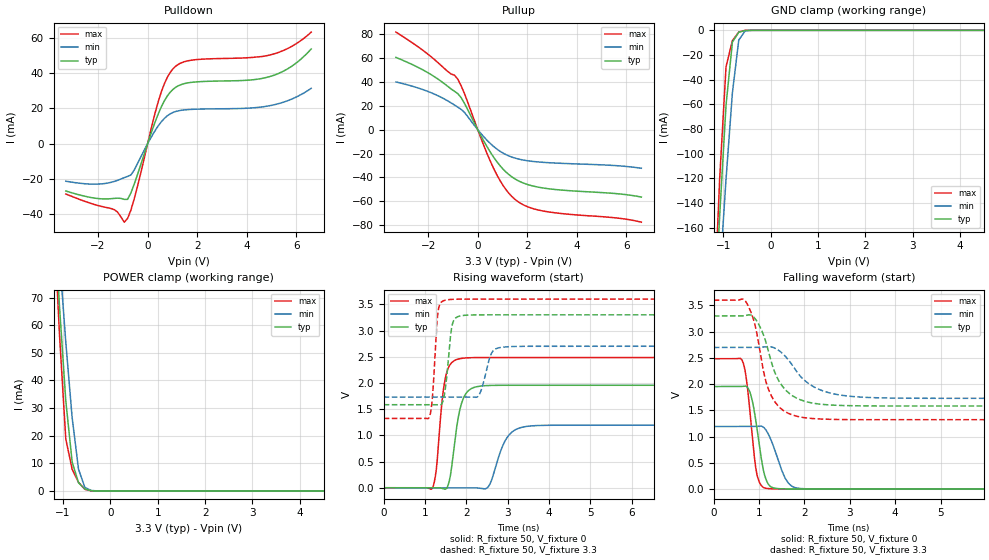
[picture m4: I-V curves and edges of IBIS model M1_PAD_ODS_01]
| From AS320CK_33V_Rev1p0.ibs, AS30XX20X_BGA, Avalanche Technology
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[Model] M1_PAD_ODS_01
Model_type I/O
Enable   Active-High
Vinl  =  0.8
Vinh  =  2.2
Vmeas =  1.65
Cref  =  30e-12
| Capacitance  typ   min   max
C_comp   1.518728e-12   1.426995e-12   1.652439e-12
| Variables   typ   min   max
[GND Clamp Reference]   0   0   0
[POWER Clamp Reference]   3.3   2.7   3.6
[Pulldown Reference]   0   0   0
[Pullup Reference]   3.3   2.7   3.6
[Temperature Range]   25   125   -40
[Voltage Range]   3.3   2.7   3.6
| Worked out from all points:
|   slope of the pulldown table from 0 to 0.495 V, typ, clamps not added: 26.1 ohm
|   slope of the pullup table from 0 to 0.495 V, typ, clamps not added: 27 ohm
|   GND clamp passes 1 mA (typ) near -0.62 V on its own axis
|   POWER clamp passes 1 mA (typ) near -0.56 V on its own axis
|   falling waveform, R_fixture 50, V_fixture 0: 20-80 % time 210ps typ, 304ps min, 176ps max; typ from 1.96 V to 0 V
|   falling waveform, R_fixture 50, V_fixture 3.3: 20-80 % time 456ps typ, 660ps min, 366ps max; typ from 3.3 V to 1.58 V
|   rising waveform, R_fixture 50, V_fixture 0: 20-80 % time 224ps typ, 335ps min, 176ps max; typ from 0 V to 1.96 V
|   rising waveform, R_fixture 50, V_fixture 3.3: 20-80 % time 128ps typ, 193ps min, 104ps max; typ from 1.58 V to 3.3 V
[GND Clamp]
| Voltage   I(typ)   I(min)   I(max)
-3.3V     -1.961A    -1.697A    -2.357A
-1.21V    -250.6mA   -283.7mA   -242.3mA
-1.076V   -150.5mA   -200.1mA   -120.5mA
-941.4mV  -60.74mA   -120.8mA   -29.57mA
-806.9mV  -9.575mA   -50.7mA    -8.297mA
-672.4mV  -1.554mA   -7.862mA   -1.403mA
-537.9mV  -68.54uA   -503.1uA   -16.86uA
-403.4mV  -562.8nA   -18.5uA    -33.35nA
6.6V      0A         0A         0A
[POWER Clamp]
| Voltage   I(typ)   I(min)   I(max)
-3.3V     772.3mA    673.3mA    930.5mA
-1.21V    105.9mA    117.6mA    104.6mA
-1.076V   67.34mA    85.06mA    57.16mA
-941.4mV  32.71mA    53.93mA    18.82mA
-806.9mV  10.48mA    26.53mA    7.848mA
-672.4mV  2.975mA    7.856mA    3.108mA
-537.9mV  710.9uA    1.248mA    573.1uA
-403.4mV  60.69uA    160.8uA    9.187uA
-269mV    142.4nA    6.118uA    23.26nA
6.6V      0A         0A         0A
[Pulldown]
| Voltage   I(typ)   I(min)   I(max)
-3.3V     -26.75mA   -21.23mA   -28.47mA
-1.345V   -30.95mA   -21.36mA   -37.3mA
-941.4mV  -31.51mA   -19.19mA   -44.41mA
-806.9mV  -31.48mA   -18.5mA    -42.27mA
-537.9mV  -22.81mA   -14.83mA   -31.1mA
455.2mV   17.74mA    10.61mA    25.04mA
682.8mV   24.44mA    14.41mA    34.16mA
1.024V    30.75mA    17.67mA    42.38mA
1.821V    34.78mA    19.45mA    47.35mA
4.914V    37.93mA    21.47mA    50.14mA
5.783V    43.54mA    25.06mA    54.82mA
6.6V      53.61mA    31.34mA    63.15mA
[Pullup]
| Voltage   I(typ)   I(min)   I(max)
-3.3V     60.72mA    40.13mA    81.98mA
-1.883V   46.28mA    31.07mA    61.29mA
-806.9mV  30.37mA    18.97mA    42.5mA
-537.9mV  22.23mA    14.55mA    30.47mA
227.6mV   -8.879mA   -5.576mA   -12.4mA
682.8mV   -24.3mA    -14.8mA    -34.27mA
1.138V    -35.52mA   -20.92mA   -50.3mA
1.593V    -42.39mA   -24.36mA   -59.94mA
2.048V    -46.27mA   -26.18mA   -65mA
2.731V    -49.23mA   -27.53mA   -68.61mA
5.659V    -53.82mA   -30.29mA   -74.27mA
6.6V      -56.57mA   -32.36mA   -77.67mA
[Ramp]
dV/dt_r   1.17342/0.223753n  0.716081/0.335063n  1.491/0.176015n
dV/dt_f   1.02933/0.456193n  0.581576/0.660479n  1.3662/0.365831n
R_load = 50
[Falling Waveform]
R_fixture = 50
V_fixture = 0
V_fixture_min = 0
V_fixture_max = 0
| Time   V(typ)   V(min)   V(max)
0s        1.956V     1.193V     2.485V
633.4ps   1.958V     1.194V     2.44V
712ps     1.961V     1.194V     2.14V
795.4ps   1.851V     1.194V     1.501V
937ps     1.251V     1.196V     345.3mV
1.077ns   436.5mV    1.191V     42.26mV
1.183ns   125.1mV    1.081V     12.58mV
1.587ns   4.061mV    190.6mV    1.4mV
1.937ns   1.085mV    10.77mV    405.9uV
21.88ns   -318.8nV   -148.1nV   831.4nV
[Falling Waveform]
R_fixture = 50
V_fixture = 3.3
V_fixture_min = 2.7
V_fixture_max = 3.6
| Time   V(typ)   V(min)   V(max)
0s        3.3V       2.7V       3.6V
697.8ps   3.307V     2.7V       3.585V
872.4ps   3.286V     2.701V     3.244V
983ps     3.153V     2.701V     2.809V
1.133ns   2.85V      2.714V     2.108V
1.264ns   2.442V     2.711V     1.788V
1.542ns   1.931V     2.564V     1.494V
1.988ns   1.68V      2.083V     1.363V
3.639ns   1.585V     1.74V      1.324V
21.88ns   1.584V     1.731V     1.323V
[Rising Waveform]
R_fixture = 50
V_fixture = 0
V_fixture_min = 0
V_fixture_max = 0
| Time   V(typ)   V(min)   V(max)
0s        8.005nV    63.52nV    4.761nV
1.177ns   816.1uV    -403.8uV   -9.581mV
1.274ns   883.4uV    -437.1uV   350.1mV
1.496ns   -26.27mV   -513.1uV   2.104V
1.603ns   180.5mV    -549.8uV   2.345V
1.893ns   1.629V     -649.3uV   2.47V
2.507ns   1.95V      -1.089mV   2.485V
2.994ns   1.955V     964.9mV    2.485V
3.586ns   1.955V     1.181V     2.485V
21.88ns   1.956V     1.193V     2.485V
[Rising Waveform]
R_fixture = 50
V_fixture = 3.3
V_fixture_min = 2.7
V_fixture_max = 3.6
| Time   V(typ)   V(min)   V(max)
0s        1.584V     1.731V     1.323V
1.099ns   1.585V     1.731V     1.338V
1.176ns   1.585V     1.731V     1.686V
1.318ns   1.586V     1.731V     3.373V
1.447ns   1.689V     1.731V     3.568V
1.551ns   2.319V     1.731V     3.588V
1.686ns   3.175V     1.732V     3.596V
2.001ns   3.293V     1.732V     3.599V
2.996ns   3.299V     2.69V      3.599V
21.88ns   3.3V       2.7V       3.6V
